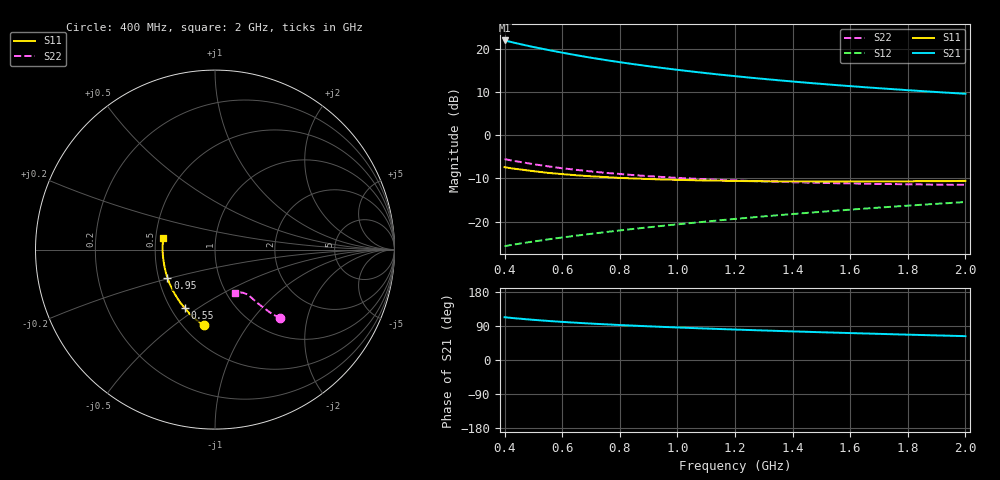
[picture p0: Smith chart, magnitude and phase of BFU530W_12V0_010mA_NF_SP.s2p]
! Filename:  P:\Prog\Test\Noise\ATS_data\Testdata_Net\06 Compressed Noise after Statistics\BFU530W_APM2013_09_A05_12p0V_010mA_NF_CM01_D.sf
! Date/Time: Tue 26/Mar/2013 18:06:01
! BFU530W_APM2013_09_A05_12p0V_1to25mA_NF_CM01_Bias6_R.sf
! Noise Parameter Data File
! BFU530W_APM2013_09_A05_12p0V_1to25mA_NF_CM01
! Date/time: Thu Mar 21 22:54:15 2013
! VAR V_out= 12.000000
! VAR I_out= 9.990000
! VAR V_in= 0.797300
! VAR I_in= 0.088705
! Device data file deembeded for feedlines and parallel
! Original file: \06 Compressed Noise after Statistics\BFU530W_APM2013_09_A05_12p0V_010mA_NF_CM01_R.sf
! Feed-files: PR019V01_070313_Feed1.s2p, PR019V01_070313_Feed2.s2p
! Parallel-file: PR019V01_070313_Par.s2p
# MHz S MA R 50
!  Freq-MHz  S11-mag  S11-arg  S21-mag  S21-arg  S12-mag  S12-arg  S22-mag  S22-arg
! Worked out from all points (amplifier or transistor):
!   37 points, 400 MHz to 2 GHz, reference 50 ohm
!   highest |S21| = 21.9 dB at 400 MHz (marker M1)
!   |S21| within 3 dB of that: start of sweep to 615 MHz
!   unconditionally stable (mu >= 1): 1.475 GHz to end of sweep
!   at 500 MHz: K = 0.71, MSG = 22.5 dB, |S12| = -24.6 dB
!   at 1.1 GHz: K = 0.96, MSG = 17.1 dB, |S12| = -20.0 dB
!   at 2 GHz: K = 1.02, MAG = 11.7 dB, |S12| = -15.5 dB
!   lowest NFmin = 0.76 dB at 420 MHz
!   S11 on the Smith chart (normalised r, x): 400 MHz: 0.63, -0.65; 550 MHz: 0.59, -0.44; 950 MHz: 0.56, -0.19; 2 GHz: 0.55, +0.08
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400  0.4261 -98.5  12.41 112.8  0.05217 59.1  0.5284 -46.3
420  0.4161 -101.4  11.97 111.3  0.05363 59.0  0.5134 -47.0
440  0.407 -104.1  11.55 109.9  0.055 59.0  0.4992 -47.5
480  0.3913 -109.2  10.78 107.2  0.05772 59.0  0.4742 -48.5
500  0.3839 -111.8  10.43 106.0  0.05903 59.1  0.4621 -48.9
550  0.3667 -117.2  9.66 103.1  0.06239 59.4  0.4366 -49.7
600  0.3549 -122.5  8.974 100.6  0.06577 59.8  0.4146 -50.3
650  0.3437 -127.1  8.373 98.3  0.06907 60.1  0.397 -50.9
700  0.3348 -131.6  7.846 96.1  0.07244 60.5  0.3812 -51.4
750  0.3278 -135.6  7.377 94.2  0.07583 60.9  0.3671 -51.7
800  0.3205 -139.5  6.963 92.3  0.0793 61.3  0.3562 -52.2
850  0.316 -143.2  6.593 90.5  0.08273 61.7  0.345 -52.5
950  0.3071 -149.6  5.958 87.3  0.08975 62.4  0.3284 -53.3
1050  0.3019 -155.4  5.434 84.4  0.09681 62.9  0.315 -54.0
1150  0.2977 -160.9  4.994 81.7  0.1041 63.3  0.3039 -54.7
1200  0.2956 -163.2  4.805 80.4  0.1078 63.5  0.3002 -55.3
1250  0.2944 -165.7  4.624 79.1  0.1114 63.6  0.2956 -55.6
1350  0.2928 -169.9  4.309 76.7  0.119 63.8  0.2894 -56.6
1500  0.2917 -176.1  3.908 73.2  0.1302 63.9  0.2812 -58.4
1650  0.2918 178.2  3.58 70.0  0.1416 63.8  0.275 -60.1
1750  0.2927 175.0  3.396 67.9  0.1494 63.7  0.2723 -61.4
2000  0.2967 167.2  3.007 62.9  0.1688 63.1  0.2669 -65.2
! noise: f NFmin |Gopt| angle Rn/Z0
400  0.8106  0.04423  131.9  0.0949
460  0.7957  0.05087  134.4  0.0958
600  0.8408  0.05355  143  0.095
800  0.8664  0.08799  145.6  0.0892
1000  0.8827  0.1106  152.4  0.0857
1200  0.935  0.1321  156.8  0.0848
1400  0.935  0.1608  163.2  0.0813
1600  0.9664  0.1757  169  0.078
1800  0.9841  0.199  175.6  0.0766
2000  1.015  0.2201  -178  0.0771
